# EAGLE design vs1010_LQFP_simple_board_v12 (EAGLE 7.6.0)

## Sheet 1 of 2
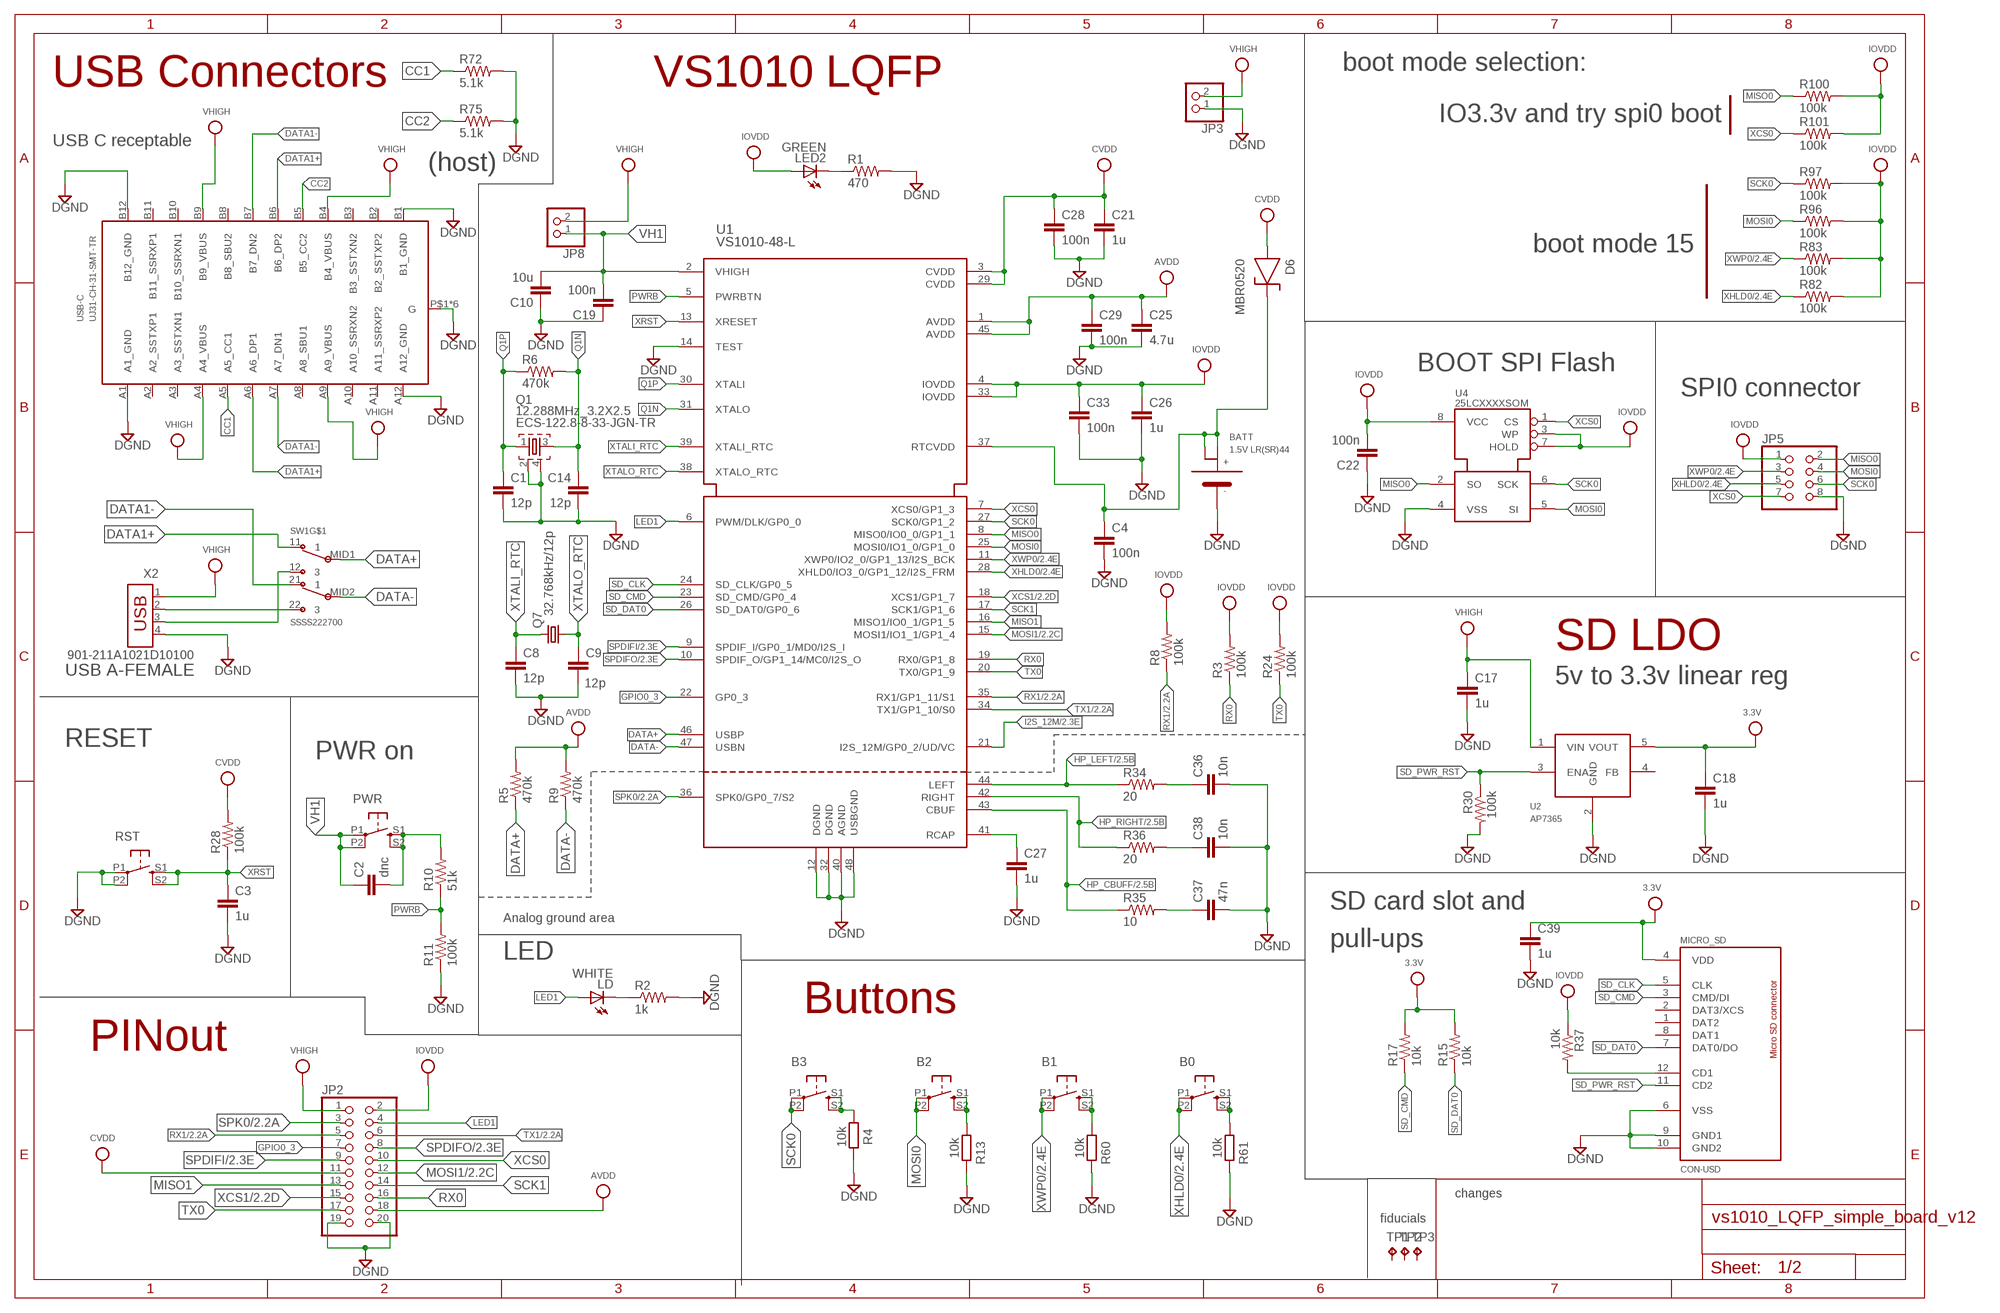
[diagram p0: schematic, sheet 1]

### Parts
B0  TS-1187A-C-E-B  SW_SMD-SW-4_5.1X5.1X2.5_TS-1187A-C-E-B_C318887  [SW_SMD-SW-4_5.1X5.1X2.5_TS-1187A-C-E-B_C318887]
B1  TS-1187A-C-E-B  SW_SMD-SW-4_5.1X5.1X2.5_TS-1187A-C-E-B_C318887  [SW_SMD-SW-4_5.1X5.1X2.5_TS-1187A-C-E-B_C318887]
B2  TS-1187A-C-E-B  SW_SMD-SW-4_5.1X5.1X2.5_TS-1187A-C-E-B_C318887  [SW_SMD-SW-4_5.1X5.1X2.5_TS-1187A-C-E-B_C318887]
B3  TS-1187A-C-E-B  SW_SMD-SW-4_5.1X5.1X2.5_TS-1187A-C-E-B_C318887  [SW_SMD-SW-4_5.1X5.1X2.5_TS-1187A-C-E-B_C318887]
BATT  1.5V LR(SR)44  BATT-LR44-TH  [KS2997]
C1  12p  C-EUC0603K  [C0603K]
C2  dnc  C-EUC0603K  [C0603K]
C3  1u  C-EUC0603K  [C0603K]
C4  100n  C-EUC0603K  [C0603K]
C8  12p  C-EUC0603K  [C0603K]
C9  12p  C-EUC0603K  [C0603K]
C10  10u  C-EUC0603K  [C0603K]
C14  12p  C-EUC0603K  [C0603K]
C17  1u  C-EUC0603K  [C0603K]
C18  1u  C-EUC0603K  [C0603K]
C19  100n  C-EUC0603K  [C0603K]
C21  1u  C-EUC0603K  [C0603K]
C22  100n  C-EUC0603K  [C0603K]
C25  4.7u  C-EUC0603K  [C0603K]
C26  1u  C-EUC0603K  [C0603K]
C27  1u  C-EUC0603K  [C0603K]
C28  100n  C-EUC0603K  [C0603K]
C29  100n  C-EUC0603K  [C0603K]
C33  100n  C-EUC0603K  [C0603K]
C36  10n  C-EUC0603K  [C0603K]
C37  47n  C-EUC0603K  [C0603K]
C38  10n  C-EUC0603K  [C0603K]
C39  1u  C-EUC0603K  [C0603K]
D6  MBR0520  [SOD-123]
JP2  PINHD-2X10  [2X10]
JP3  PINHD-1X2  [1X02]
JP5  PINHD-2X4  [2X04]
JP8  PINHD-1X2  [1X02]
LD  WHITE  LEDCHIP-LED0805  [CHIP-LED0805]
LED2  GREEN  LEDCHIP-LED0805  [CHIP-LED0805]
MICRO_SD  CON-USD  [MSSN09-A0-3000]
PWR  TS-1187A-C-E-B  SW_SMD-SW-4_5.1X5.1X2.5_TS-1187A-C-E-B_C318887  [SW_SMD-SW-4_5.1X5.1X2.5_TS-1187A-C-E-B_C318887]
Q1  12.288MHz_3.2X2.5  CRYSTAL_3.2X2.5  [3.2X2.5_CRYSTAL]
Q7  32.768kHz/12p  CRYSTAL3.2X1.5MM  [CRYSTAL_1206]
R1  470  R-US_R0603  [R0603]
R2  1k  R-US_R0603  [R0603]
R3  100k  R-US_R0603  [R0603]
R4  10k  R-EU_R0603  [R0603]
R5  470k  R-US_R0603  [R0603]
R6  470k  R-US_R0603  [R0603]
R8  100k  R-US_R0603  [R0603]
R9  470k  R-US_R0603  [R0603]
R10  51k  R-US_R0603  [R0603]
R11  100k  R-US_R0603  [R0603]
R13  10k  R-EU_R0603  [R0603]
R15  10k  R-US_R0603  [R0603]
R17  10k  R-US_R0603  [R0603]
R24  100k  R-US_R0603  [R0603]
R28  100k  R-US_R0603  [R0603]
R30  100k  R-US_R0603  [R0603]
R34  20  R-US_R0603  [R0603]
R35  10  R-US_R0603  [R0603]
R36  20  R-US_R0603  [R0603]
R37  10k  R-US_R0603  [R0603]
R60  10k  R-EU_R0603  [R0603]
R61  10k  R-EU_R0603  [R0603]
R72  5.1k  R-US_R0603  [R0603]
R75  5.1k  R-US_R0603  [R0603]
R82  100k  R-US_R0603  [R0603]
R83  100k  R-US_R0603  [R0603]
R96  100k  R-US_R0603  [R0603]
R97  100k  R-US_R0603  [R0603]
R100  100k  R-US_R0603  [R0603]
R101  100k  R-US_R0603  [R0603]
RST  TS-1187A-C-E-B  SW_SMD-SW-4_5.1X5.1X2.5_TS-1187A-C-E-B_C318887  [SW_SMD-SW-4_5.1X5.1X2.5_TS-1187A-C-E-B_C318887]
SW1  SSSS222700  SWITCH_ON-ON_DUAL_SSSS222700_C136144  [SWITCH_ON-ON_DUAL_SSSS222700_C136144]
TP1  TPTP10R  [TP10R]
TP2  TPTP10R  [TP10R]
TP3  TPTP10R  [TP10R]
U1  VS1010-48-L  [LQFP48]
U2  AP7365  [SOT23-5L]
U4  25LCXXXXSOM  [SO-8MN]
USB-C  UJ31-CH-31-SMT-TR  USB_C  [UJ31-CH-31-SMT-TR]
X2  901-211A1021D10100  USB-AH  [USB-S]

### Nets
3.3V: C18.1 C39.1 MICRO_SD.4(VDD) R15.2 R17.2 U2.5(VOUT)
AVDD: C25.1 C29.1 JP2.18 R5.2 R9.2 U1.1(AVDD) U1.45(AVDD) ; also sheet 2
CC1: R72.1 USB-C.A5(A5_CC1)
CC2: R75.1 USB-C.B5(B5_CC2)
CVDD: C21.1 C28.1 D6.ANODE JP2.11 R28.2 U1.3(CVDD) U1.29(CVDD)
DATA1+: SW1.11 USB-C.A6(A6_DP1) USB-C.B6(B6_DP2)
DATA1-: SW1.21 USB-C.A7(A7_DN1) USB-C.B7(B7_DN2)
DATA+: R5.1 SW1.MID1(MID) U1.46(USBP)
DATA-: R9.1 SW1.MID2(MID) U1.47(USBN)
DGND: BATT.NEG(-) C1.2 C3.2 C4.2 C8.2 C9.2 C10.1 C14.2 C17.2 C18.2 C19.1 C21.2 C22.1 C25.2 C26.2 C27.2 C28.2 C29.2 C33.2 C36.2 C37.2 C38.2 C39.2 JP2.19 JP2.20 JP3.1 JP5.8 MICRO_SD.6(VSS) MICRO_SD.9(GND1) MICRO_SD.10(GND2) Q1.2 Q1.4 R1.2 R2.2 R4.2 R11.1 R13.2 R30.2 R60.2 R61.2 R72.2 R75.2 RST.P1 RST.P2 U1.12(DGND) U1.14(TEST) U1.32(DGND) U1.40(AGND) U1.48(USBGND) U2.2(GND) U4.4(VSS) USB-C.A1(A1_GND) USB-C.A12(A12_GND) USB-C.B1(B1_GND) USB-C.B12(B12_GND) USB-C.P$1(G) USB-C.P$3(G) USB-C.P$4(G) USB-C.P$6(G) USB-C.P$7(G) USB-C.P$8(G) X2.4 ; also sheet 2
GPIO0_3: JP2.7 U1.22(GP0_3)
HP_CBUFF: R35.1 U1.43(CBUF) ; also sheet 2
HP_LEFT: R34.1 U1.44(LEFT) ; also sheet 2
HP_RIGHT: R36.1 U1.42(RIGHT) ; also sheet 2
I2S_12M: U1.21(I2S_12M/GP0_2/UD/VC) ; also sheet 2
IOVDD: C22.2 C26.1 C33.1 JP2.2 JP5.1 LED2.A R3.2 R8.2 R24.2 R37.1 R82.2 R83.2 R96.2 R97.2 R100.2 R101.2 U1.4(IOVDD) U1.33(IOVDD) U4.3(WP) U4.7(HOLD) U4.8(VCC) ; also sheet 2
LED1: JP2.4 LD.A U1.6(PWM/DLK/GP0_0)
MISO0: JP5.2 R100.1 U1.8(MISO0/IO0_0/GP1_1) U4.2(SO)
MISO1: JP2.13 U1.16(MISO1/IO0_1/GP1_5)
MOSI0: B2.P1 B2.P2 JP5.4 R96.1 U1.25(MOSI0/IO1_0/GP1_0) U4.5(SI)
MOSI1: JP2.12 U1.15(MOSI1/IO1_1/GP1_4) ; also sheet 2
N$2: LD.C R2.1
N$3: LED2.C R1.1
N$6: B1.S1 B1.S2 R60.1
N$9: C2.2 PWR.S1 PWR.S2 R10.2
N$10: C27.1 U1.41(RCAP)
N$17: C36.1 R34.2
N$19: C38.1 R36.2
N$20: C37.1 R35.2
N$21: MICRO_SD.12(CD1) R37.2
N$41: B0.S1 B0.S2 R61.1
N$89: B2.S1 B2.S2 R13.1
N$100: B3.S1 B3.S2 R4.1
PWRB: R10.1 R11.2 U1.5(PWRBTN)
Q1N: C14.1 Q1.3 R6.2 U1.31(XTALO)
Q1P: C1.1 Q1.1 R6.1 U1.30(XTALI)
RTCVDD: BATT.P1(+) BATT.P2(+1) C4.1 D6.CATHODE U1.37(RTCVDD)
RX0: JP2.16 R3.1 U1.19(RX0/GP1_8)
RX1: JP2.5 R8.1 U1.35(RX1/GP1_11/S1) ; also sheet 2
SCK0: B3.P1 B3.P2 JP5.6 R97.1 U1.27(SCK0/GP1_2) U4.6(SCK)
SCK1: JP2.14 U1.17(SCK1/GP1_6)
SD_CLK: MICRO_SD.5(CLK) U1.24(SD_CLK/GP0_5)
SD_CMD: MICRO_SD.3(CMD/DI) R17.1 U1.23(SD_CMD/GP0_4)
SD_DAT0: MICRO_SD.7(DAT0/DO) R15.1 U1.26(SD_DAT0/GP0_6)
SD_PWR_RST: MICRO_SD.11(CD2) R30.1 U2.3(ENA)
SPDIFI: JP2.9 U1.9(SPDIF_I/GP0_1/MD0/I2S_I) ; also sheet 2
SPDIFO: JP2.8 U1.10(SPDIF_O/GP1_14/MC0/I2S_O) ; also sheet 2
SPK0: JP2.3 U1.36(SPK0/GP0_7/S2) ; also sheet 2
TX0: JP2.17 R24.1 U1.20(TX0/GP1_9)
TX1: JP2.6 U1.34(TX1/GP1_10/S0) ; also sheet 2
USB2+: SW1.12 X2.3
USB2-: SW1.22 X2.2
VH1: C2.1 C10.2 C19.2 JP8.1 PWR.P1 PWR.P2 U1.2(VHIGH)
VHIGH: C17.1 JP2.1 JP3.2 JP8.2 U2.1(VIN) USB-C.A4(A4_VBUS) USB-C.A9(A9_VBUS) USB-C.B4(B4_VBUS) USB-C.B9(B9_VBUS) X2.1
XCS0: JP2.10 JP5.7 R101.1 U1.7(XCS0/GP1_3) U4.1(CS)
XCS1: JP2.15 U1.18(XCS1/GP1_7) ; also sheet 2
XHLD0: B0.P1 B0.P2 JP5.5 R82.1 U1.28(XHLD0/IO3_0/GP1_12/I2S_FRM) ; also sheet 2
XRST: C3.1 R28.1 RST.S1 RST.S2 U1.13(XRESET)
XTALI_RTC: C8.1 Q7.2 U1.39(XTALI_RTC)
XTALO_RTC: C9.1 Q7.1 U1.38(XTALO_RTC)
XWP0: B1.P1 B1.P2 JP5.3 R83.1 U1.11(XWP0/IO2_0/GP1_13/I2S_BCK) ; also sheet 2
Unconnected: MICRO_SD.1(DAT2) MICRO_SD.2(DAT3/XCS) MICRO_SD.8(DAT1) TP1.TP TP2.TP TP3.TP U2.4(FB) USB-C.A2(A2_SSTXP1) USB-C.A3(A3_SSTXN1) USB-C.A8(A8_SBU1) USB-C.A10(A10_SSRXN2) USB-C.A11(A11_SSRXP2) USB-C.B2(B2_SSTXP2) USB-C.B3(B3_SSTXN2) USB-C.B8(B8_SBU2) USB-C.B10(B10_SSRXN1) USB-C.B11(B11_SSRXP1)

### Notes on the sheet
- USB Connectors | VS1010 LQFP | boot mode selection:
- IO3.3v and try spi0 boot
- USB C receptable
- (host)
- boot mode 15
- BOOT SPI Flash
- SPI0 connector
- SD LDO
- USB A-FEMALE
- 5v to 3.3v linear reg
- RESET
- PWR on
- SD card slot and
- Analog ground area
- pull-ups
- LED
- Buttons
- PINout
- changes
- fiducials

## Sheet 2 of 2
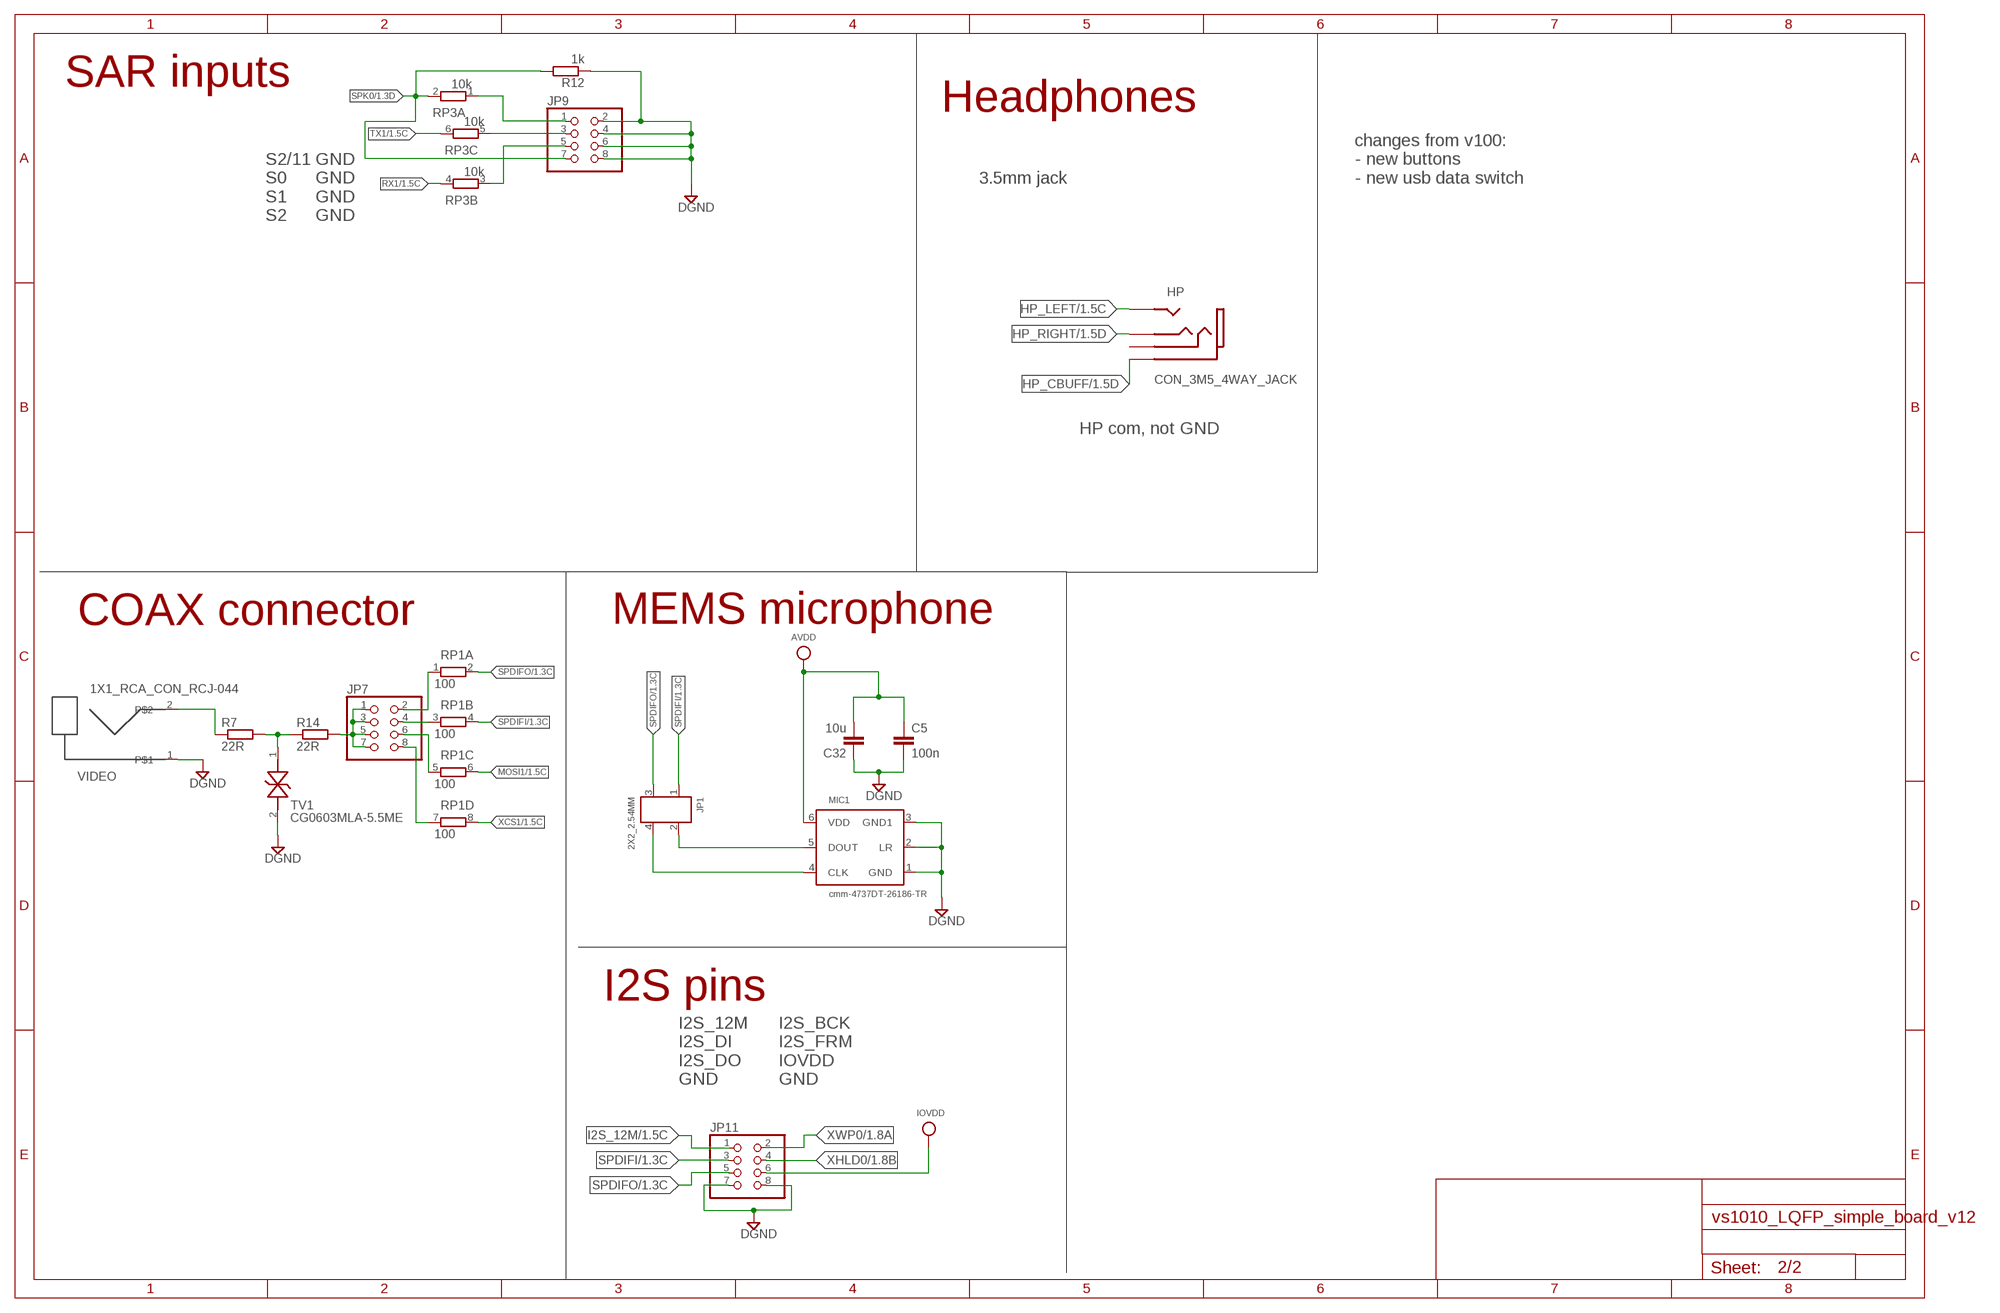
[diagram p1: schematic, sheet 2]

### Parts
C5  100n  C-EUC0603K  [C0603K]
C32  10u  C-EUC0805  [C0805]
HP  CON_3M5_4WAY_JACK  CON_3M5_4WAY_JACK-TH  [SJ-43514]
JP1  2X2_2.54MM  2X2_2.54MM_CON_THRU  [2X2_2.54MM_CON_THRU]
JP7  PINHD-2X4  [2X04]
JP9  PINHD-2X4  [2X04]
JP11  PINHD-2X4  [2X04]
MIC1  cmm-4737DT-26186-TR  MEMS_MIC_CMM-4737DT-26186-TR  [MIC_MEMS_CMM-4737DT]
R7  22R  R-EU_R0603  [R0603]
R12  1k  R-EU_R0603  [R0603]
R14  22R  R-EU_R0603  [R0603]
RP1  100  RESPAK-4X1206  [RAS_ARR_1206]
RP3  10k  RESPAK-4X1206  [RAS_ARR_1206]
TV1  CG0603MLA-5.5ME  [0603]
VIDEO  1X1_RCA_CON_RCJ-044  [1X1_RCA_CON_RCJ-044]

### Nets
AVDD: C5.1 C32.2 MIC1.6(VDD) ; also sheet 1
DGND: C5.2 C32.1 JP9.2 JP9.4 JP9.6 JP9.8 JP11.7 JP11.8 MIC1.1(GND) MIC1.2(LR) MIC1.3(GND1) R12.1 TV1.2(A2) VIDEO.1 ; also sheet 1
HP_CBUFF: HP.5(GND) ; also sheet 1
HP_LEFT: HP.4(LEFT) ; also sheet 1
HP_RIGHT: HP.1(RIGHT) ; also sheet 1
I2S_12M: JP11.1 ; also sheet 1
IOVDD: JP11.6 ; also sheet 1
MOSI1: RP1.6 ; also sheet 1
N$5: JP9.3 RP3.5
N$7: JP9.5 RP3.3
N$8: JP1.2 MIC1.5(DOUT)
N$11: JP1.4 MIC1.4(CLK)
N$12: JP7.2 RP1.1
N$13: JP7.6 RP1.5
N$14: JP7.1 JP7.3 JP7.5 JP7.7 R14.2
N$15: JP7.4 RP1.3
N$16: JP7.8 RP1.7
N$18: R7.1 VIDEO.2
N$25: JP9.1 RP3.1
N$52: R7.2 R14.1 TV1.1(A1)
RX1: RP3.4 ; also sheet 1
SPDIFI: JP1.1 JP11.3 RP1.4 ; also sheet 1
SPDIFO: JP1.3 JP11.5 RP1.2 ; also sheet 1
SPK0: JP9.7 R12.2 RP3.2 ; also sheet 1
TX1: RP3.6 ; also sheet 1
XCS1: RP1.8 ; also sheet 1
XHLD0: JP11.4 ; also sheet 1
XWP0: JP11.2 ; also sheet 1
Unconnected: HP.6(POLE4) RP3.7 RP3.8

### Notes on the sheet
- SAR inputs
- Headphones
- 3.5mm jack
- changes from v100:
  - new buttons
  - new usb data switch
- S2/11
  S0   
  S1
  S2
- GND
  GND
  GND
  GND
- HP com, not GND
- COAX connector | MEMS microphone
- I2S pins
- I2S_12M 
  I2S_DI    
  I2S_DO 
  GND
- I2S_BCK
  I2S_FRM
  IOVDD
  GND

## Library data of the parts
B0 B1-B3 PWR RST = 121_PanunKomponentit:SW_SMD-SW-4_5.1X5.1X2.5_TS-1187A-C-E-B_C318887
BATT = Omat:BATT-LR44
C1-C5 C8-C10 C14 C17-C19 C21 C22 C25-C29 C33 C36-C39 = resistor:C-EU: CAPACITOR, European symbol
C32 = rcl:C-EU: CAPACITOR, European symbol
D6 = 121_PanunKomponentit:MBR0520
HP = Samin_e7:CON_3M5_4WAY_JACK
JP1 = 121_PanunKomponentit:2X2_2.54MM_CON_THRU
JP2 = pinhead:PINHD-2X10: PIN HEADER
JP3 JP8 = pinhead:PINHD-1X2: PIN HEADER
JP5 JP7 JP9 JP11 = pinhead:PINHD-2X4: PIN HEADER
LD LED2 = led:LED: LED
MIC1 = 121_PanunKomponentit:MEMS_MIC_CMM-4737DT-26186-TR
MICRO_SD = 114SaminOmat:CON-USD: Micro SD connector
Q1 = 121_PanunKomponentit:CRYSTAL_3.2X2.5
Q7 = antimode_x4:CRYSTAL: CRYSTAL
R1-R3 R5 R6 R8-R11 R15 R17 R24 R28 R30 R34-R37 R72 R75 R82 R83 R96 R97 R100 R101 = resistor:R-US_: RESISTOR, American symbol
R4 R7 R12-R14 R60 R61 = rcl:R-EU_: RESISTOR, European symbol
RP1 RP3 = Samin_e7:RESPAK-4X1206
SW1 = 121_PanunKomponentit:SWITCH_ON-ON_DUAL_SSSS222700_C136144
TP1-TP3 = testpad:TP: Test pad
TV1 = SaminOmat:CG0603MLA-5.5ME: Transient voltage suppressor
U1 = 121_PanunKomponentit:VS1010-48
U2 = HannunOmat:AP7365
U4 = 121_PanunKomponentit:25LCXXXX
USB-C = 121_PanunKomponentit:USB_C
VIDEO = 121_PanunKomponentit:1X1_RCA_CON_RCJ-044
X2 = SaminOmat:USB-A: AMP connector

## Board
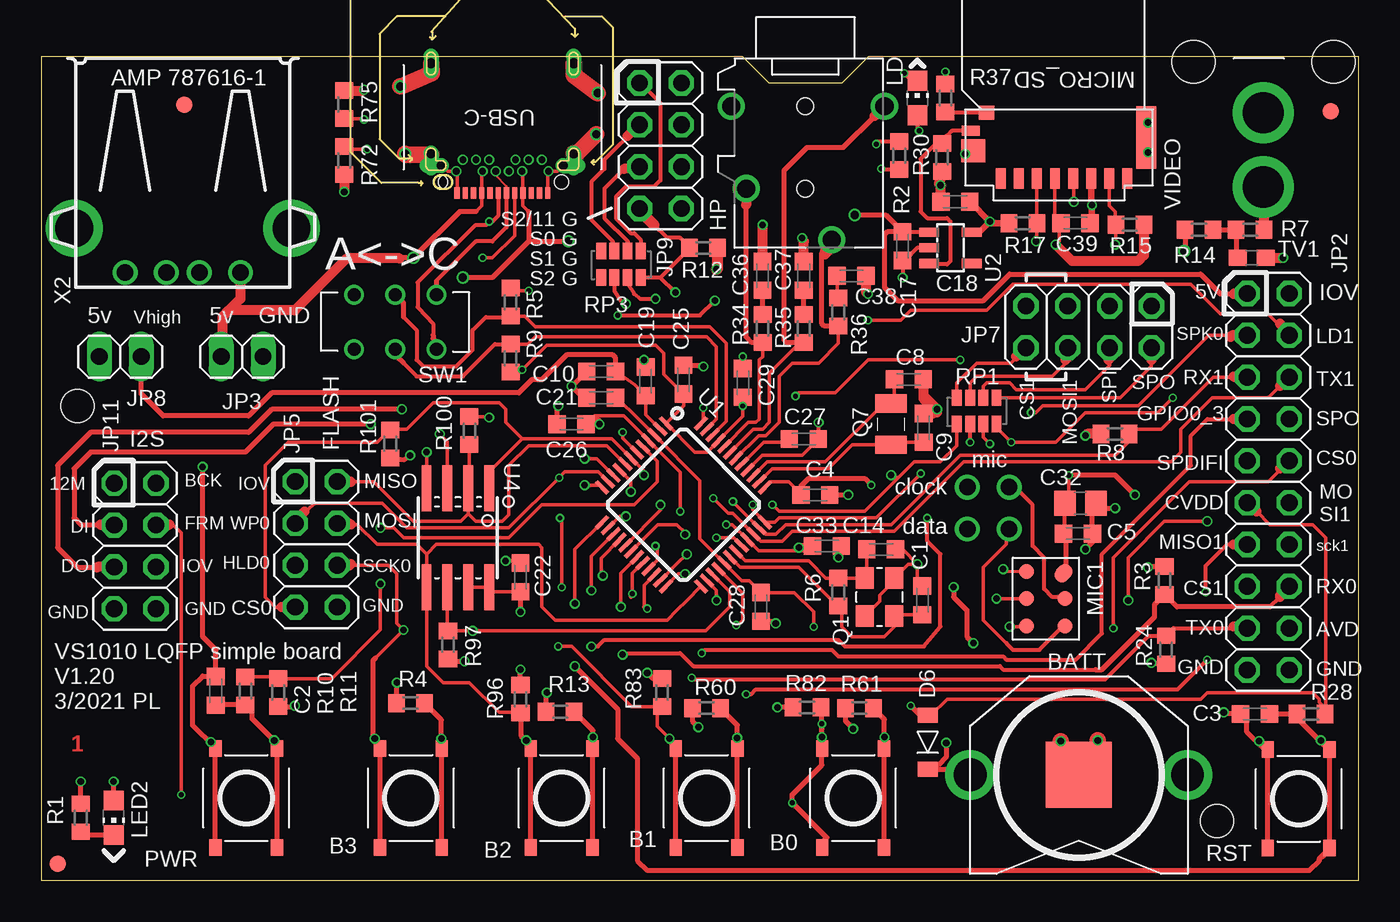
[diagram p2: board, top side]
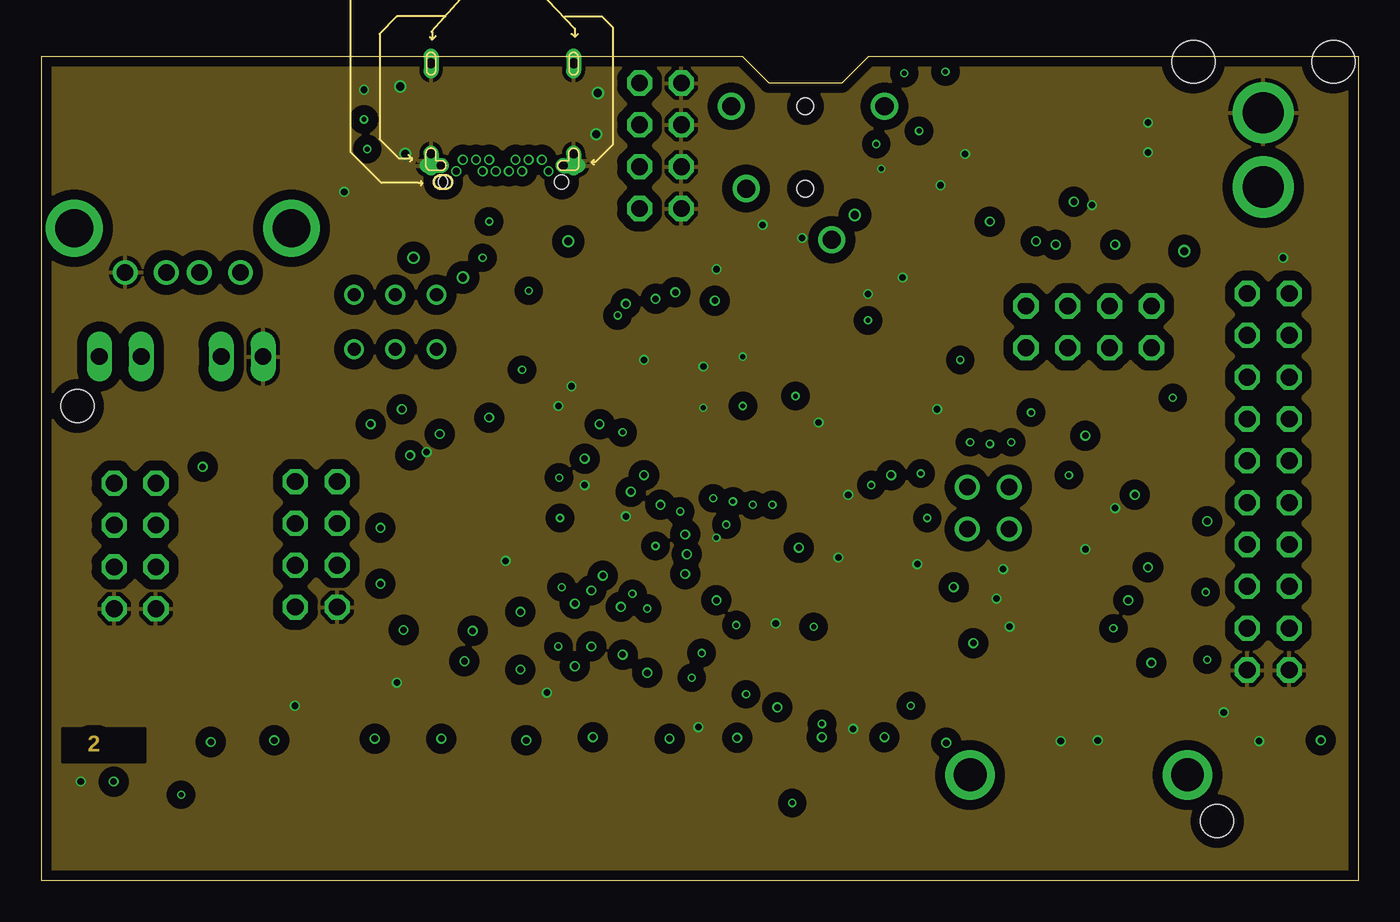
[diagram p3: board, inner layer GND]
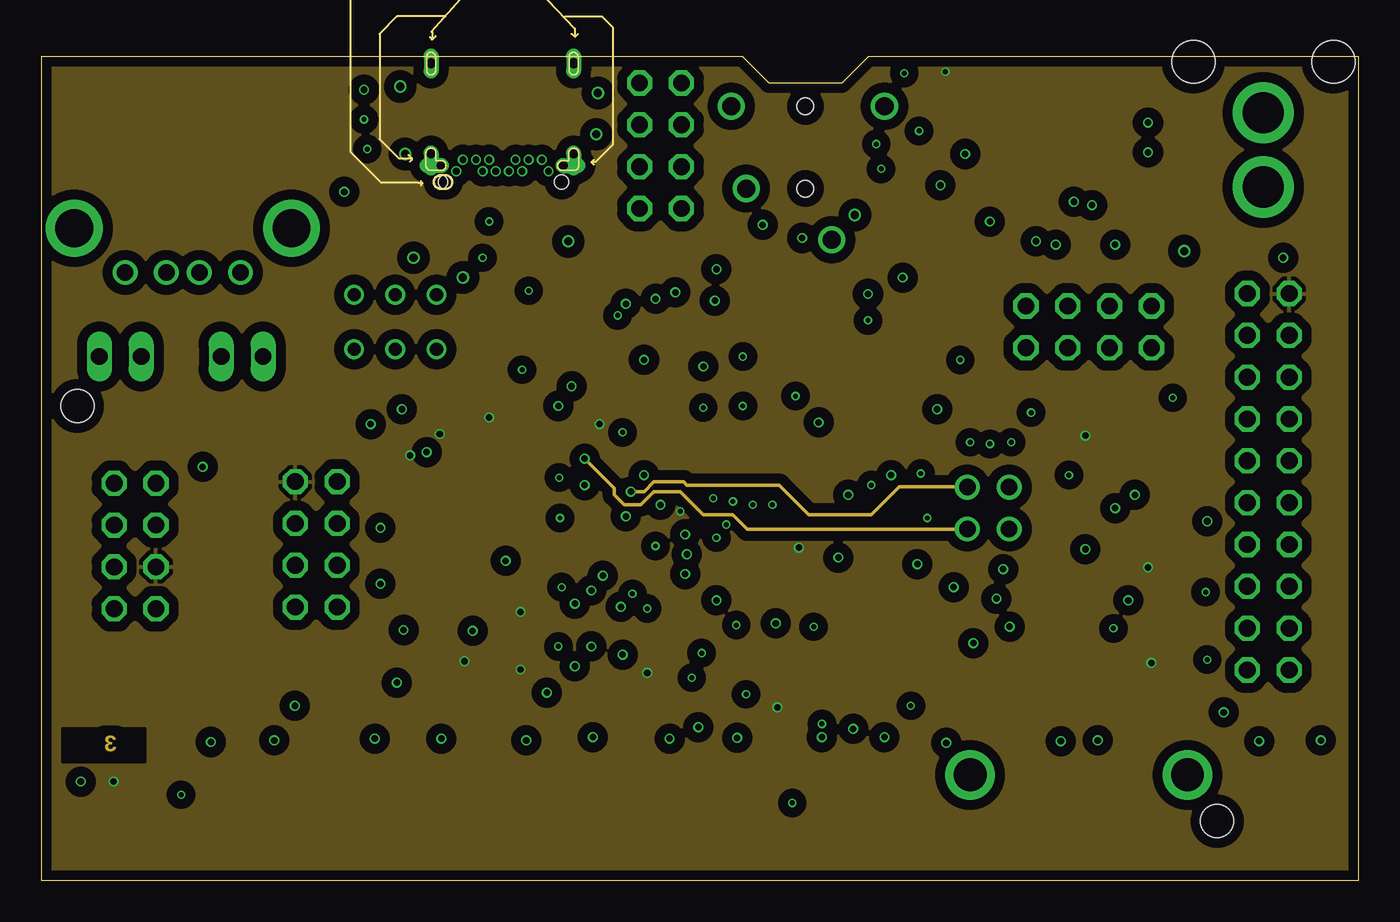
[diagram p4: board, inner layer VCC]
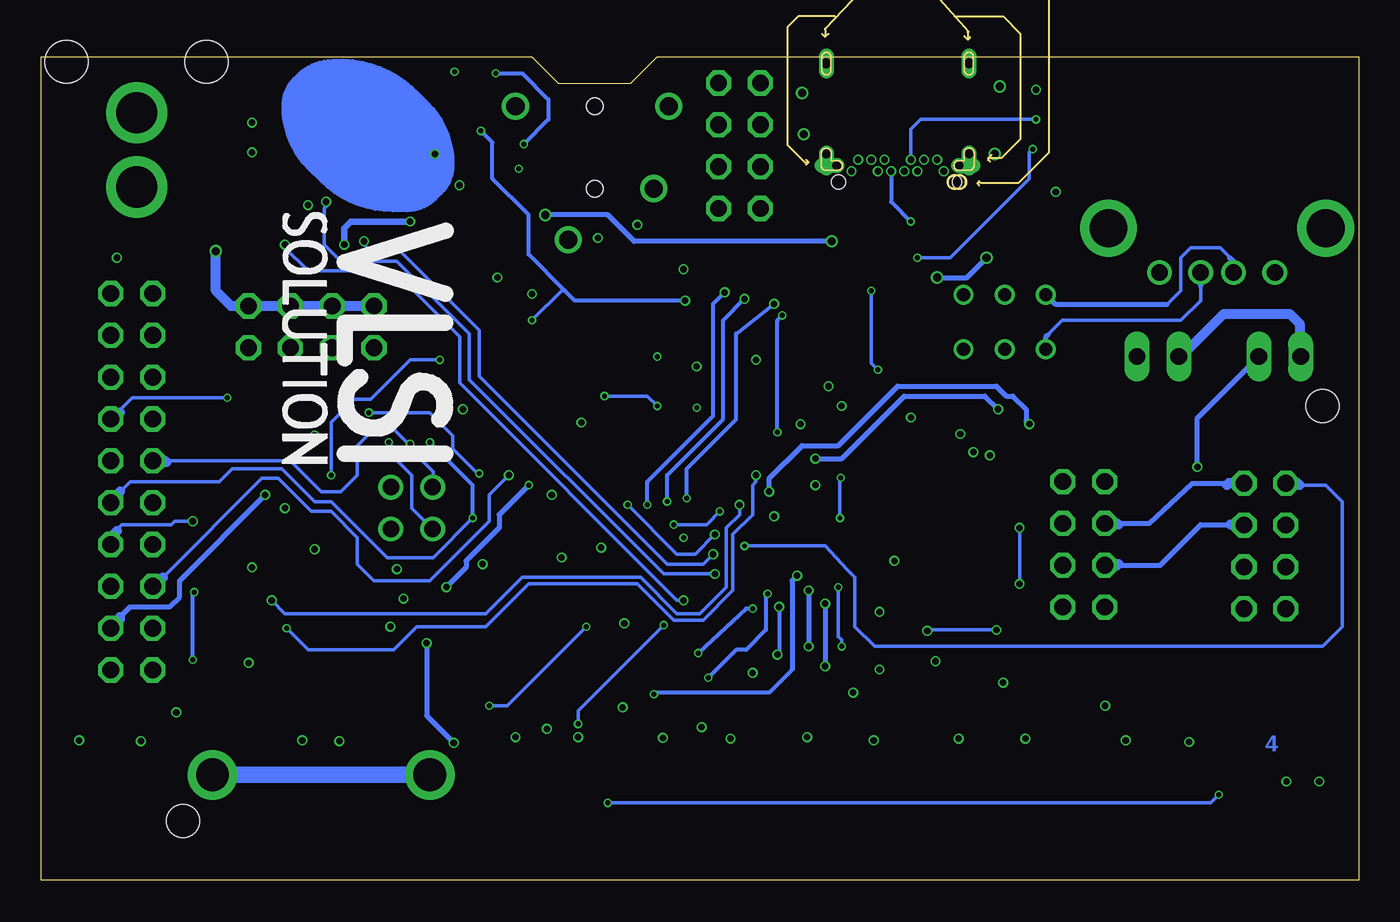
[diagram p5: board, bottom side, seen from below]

Size 80 x 50 mm. Coordinates in mm from the lower left corner, seen from the top.
Outline: 0,0 80,0 80,50 50.2,50 48.6,48.4 44.2,48.4 42.6,50 0,50 0,0
Copper layers (1*2+15*16): Top 0.035mm / dielectric 0.12mm / GND 0.0175mm / dielectric 1.2mm / VCC 0.0175mm / dielectric 0.12mm / Bottom 0.035mm
Design rules "4L_Smart_prototyping_usb-c_Eagle Rule": minimum track width 6mil, minimum drill 0.3mm, track to track 6mil, track to pad 6mil, pad to pad 6mil, via to via 6mil, smd to smd 0mil, copper to edge 6mil, drill to drill 12mil, minimum pad ring 0.1mm, minimum via ring 4mil, stop-mask expansion 2mil, vias tented up to drill 25mil, thermal gap 10mil
Holes 2 mm at 2.2,28.8 71.4,3.6

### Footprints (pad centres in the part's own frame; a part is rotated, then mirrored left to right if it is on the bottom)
SW_SMD-SW-4_5.1X5.1X2.5_TS-1187A-C-E-B_C318887 = smd 1 x 0.75: P1 -3,1.875; P2 3,1.875; S1 -3,-1.875; S2 3,-1.875
KS2997 = smd 4 x 4: NEG 0,0 | drill 2: P1 -6.6,0; P2 6.6,0
C0603K = smd 1.05 x 1.08: 1 -0.875,0; 2 0.875,0
C0805 = smd 1.3 x 1.5: 1 -0.95,0; 2 0.95,0
SOD-123 = smd 0.914 x 1.219: ANODE -1.638,0; CATHODE 1.638,0
SJ-43514 = drill 1.1: 1 8.1,1.6; 4 5,-3.6; 5 0,4.8; 6 0,-4.5 | hole 1: 0,0; 5,0
2X2_2.54MM_CON_THRU = drill 1: 1 -1.27,1.27; 2 1.27,1.27; 3 -1.27,-1.27; 4 1.27,-1.27
2X10 = drill 1.016 octagon: 1 -11.43,-1.27; 2 -11.43,1.27; 3 -8.89,-1.27; 4 -8.89,1.27; 5 -6.35,-1.27; 6 -6.35,1.27; 7 -3.81,-1.27; 8 -3.81,1.27; 9 -1.27,-1.27; 10 -1.27,1.27; 11 1.27,-1.27; 12 1.27,1.27; 13 3.81,-1.27; 14 3.81,1.27; 15 6.35,-1.27; 16 6.35,1.27; 17 8.89,-1.27; 18 8.89,1.27; 19 11.43,-1.27; 20 11.43,1.27
1X02 = drill 1.016 long: 1 -1.27,0; 2 1.27,0
2X04 = drill 1.016 octagon: 1 -3.81,-1.27; 2 -3.81,1.27; 3 -1.27,-1.27; 4 -1.27,1.27; 5 1.27,-1.27; 6 1.27,1.27; 7 3.81,-1.27; 8 3.81,1.27
CHIP-LED0805 = smd 1.2 x 1.2: A 0,-1.05; C 0,1.05
MIC_MEMS_CMM-4737DT = smd 0.91 x 0.91: 1 -1.17,1.65; 2 -1.17,0; 3 -1.17,-1.65; 4 1.17,-1.65; 5 1.17,0 | smd 1.2 x 0.91 rotated 45: 6 1.07,1.55
MSSN09-A0-3000 = smd 0.6 x 1.25: 1 3.85,0; 2 2.75,0; 3 1.65,0; 4 0.55,0; 5 -0.55,0; 6 -1.65,0; 7 -2.75,0; 8 -3.85,0 | smd 1.2 x 3.79: 9 -5,-2.5 | smd 1.45 x 1.4: 10 5.5,-1.7 | smd 1.1 x 0.6: 11 5.65,-2.9 | smd 0.95 x 0.85: 12 4.7,-4
3.2X2.5_CRYSTAL = smd 1.3 x 1.1: 1 -1.15,-0.9; 2 1.15,-0.9; 3 1.15,0.9; 4 -1.15,0.9
CRYSTAL_1206 = smd 1.1 x 1.9: 1 -1.25,0; 2 1.25,0
R0603 = smd 1 x 1.1: 1 -0.85,0; 2 0.85,0
RAS_ARR_1206 = smd 1 x 0.6: 1 -0.8,1.2; 2 0.8,1.2; 3 -0.8,0.4; 4 0.8,0.4; 5 -0.8,-0.4; 6 0.8,-0.4; 7 -0.8,-1.2; 8 0.8,-1.2
SWITCH_ON-ON_DUAL_SSSS222700_C136144 = drill 0.8: 11 -2.5,-1.65; 12 2.5,-1.65; 21 -2.5,1.65; 22 2.5,1.65; MID1 0,-1.65; MID2 0,1.65
TP10R = smd 1 x 1: TP 0,0
0603 = smd 1.1 x 1: 1 -0.85,0; 2 0.85,0
LQFP48 = smd 0.25 x 1: 1 -2.75,-4.25; 2 -2.25,-4.25; 3 -1.75,-4.25; 4 -1.25,-4.25; 5 -0.75,-4.25; 6 -0.25,-4.25; 7 0.25,-4.25; 8 0.75,-4.25; 9 1.25,-4.25; 10 1.75,-4.25; 11 2.25,-4.25; 12 2.75,-4.25; 25 2.75,4.25; 26 2.25,4.25; 27 1.75,4.25; 28 1.25,4.25; 29 0.75,4.25; 30 0.25,4.25; 31 -0.25,4.25; 32 -0.75,4.25; 33 -1.25,4.25; 34 -1.75,4.25; 35 -2.25,4.25; 36 -2.75,4.25 | smd 1 x 0.25: 13 4.25,-2.75; 14 4.25,-2.25; 15 4.25,-1.75; 16 4.25,-1.25; 17 4.25,-0.75; 18 4.25,-0.25; 19 4.25,0.25; 20 4.25,0.75; 21 4.25,1.25; 22 4.25,1.75; 23 4.25,2.25; 24 4.25,2.75; 37 -4.25,2.75; 38 -4.25,2.25; 39 -4.25,1.75; 40 -4.25,1.25; 41 -4.25,0.75; 42 -4.25,0.25; 43 -4.25,-0.25; 44 -4.25,-0.75; 45 -4.25,-1.25; 46 -4.25,-1.75; 47 -4.25,-2.25; 48 -4.25,-2.75
SOT23-5L = smd 0.55 x 1.2: 1 -0.95,-1.3; 2 0,-1.3; 3 0.95,-1.3; 4 0.95,1.3; 5 -0.95,1.3
SO-8MN = smd 0.6 x 2.8: 1 -1.905,-3.013; 2 -0.635,-3.013; 3 0.635,-3.013; 4 1.905,-3.013; 5 1.905,3.013; 6 0.635,3.013; 7 -0.635,3.013; 8 -1.905,3.013
UJ31-CH-31-SMT-TR = smd 0.32 x 0.7: A1 -2.75,0.66; A2 -2.25,0.66; A3 -1.75,0.66; A4 -1.25,0.66; A5 -0.75,0.66; A6 -0.25,0.66; A7 0.25,0.66; A8 0.75,0.66; A9 1.25,0.66; A10 1.75,0.66; A11 2.25,0.66; A12 2.75,0.66 | drill 0.4 pad 0.6: B1 2.8,-0.65; B2 2.4,-1.35; B3 1.6,-1.35; B4 1.2,-0.65; B5 0.8,-1.35; B6 0.4,-0.65; B7 -0.4,-0.65; B8 -0.8,-1.35; B9 -1.2,-0.65; B10 -1.6,-1.35; B11 -2.4,-1.35; B12 -2.8,-0.65 | drill 0.6 pad 0.8 offset: P$1 -3.68,-1; P$3 -4.33,-1.75; P$4 3.68,-1; P$6 4.33,-1.75 | drill 0.6 pad 0.9 long: P$7 -4.33,-7.2; P$8 4.33,-7.2 | hole 0.85: 3.45,0; -3.6,0; 3.75,0
1X1_RCA_CON_RCJ-044 = drill 2.5: 1 -4,0; 2 -8.5,0 | hole 2.6: -0.9,4.25; -0.9,-4.25
USB-S = drill 1: 1 -3.5,12.99; 2 -1,12.99; 3 1,12.99; 4 3.5,12.99 | drill 2.3: P$1 -6.6,10.3; P$2 6.6,10.3

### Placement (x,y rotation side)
B0  49.3,5 90 top
B1  40.4,5 90 top
B2  31.6,5 90 top
B3  22.45,5 90 top
BATT  63,6.4 180 top
C1  53.5,17 90 top
C2  10.6,11.5 270 top
C3  73.7,10.1 180 top
C4  47,23.4 0 top
C5  62.95,21.05 0 top
C8  52.68,30.42 0 top
C9  53.58,27.47 90 top
C10  34,30.9 0 top
C14  51,20.1 0 top
C17  52.3,38.5 270 top
C18  55.5,41.2 180 top
C19  36.7,30.3 270 top
C21  34,29.3 180 top
C22  29.1,18.4 270 top
C25  39,30.4 90 top
C26  32.2,27.7 180 top
C27  46.3,26.8 0 top
C28  43.7,16.6 270 top
C29  42.6,30.2 90 top
C32  63.1,22.9 180 top
C33  47.7,20.3 0 top
C36  43.8,36.7 90 top
C37  46.3,36.7 90 top
C38  49.2,36.7 0 top
C39  62.8,39.9 0 top
D6  53.83,8.38 270 top
HP  46.4,47 270 top
JP1  57.5,22.6 0 top
JP2  74.5,24.2 270 top
JP3  12.2,31.8 180 top
JP5  16.7,20.4 270 top
JP7  63.6,33.6 180 top
JP8  4.8,31.8 180 top
JP9  37.6,44.6 270 top
JP11  5.7,20.3 270 top
LD  53.2,47.5 0 top
LED2  4.4,3.8 180 top
MIC1  61,17.1 0 top
MICRO_SD  62.1,42.6 180 top
PWR  12.45,5 90 top
Q1  50.9,17.2 90 top
Q7  51.59,27.7 90 top
R1  2.4,3.8 90 top
R2  52.1,44 270 top
R3  68.2,18.2 90 top
R4  22.43,10.76 180 top
R5  28.5,35.1 90 top
R6  48.4,17.5 90 top
R7  73.4,39.5 180 top
R8  65.2,27.1 180 top
R9  28.5,31.7 270 top
R10  12.4,11.5 270 top
R11  14.4,11.4 90 top
R12  40.2,38.4 180 top
R13  31.51,10.24 180 top
R14  70.3,39.5 180 top
R15  66.1,39.8 0 top
R17  59.6,39.9 180 top
R24  68.3,14 270 top
R28  77.1,10.1 0 top
R30  54.7,43.9 270 top
R34  43.8,33.5 90 top
R35  46.3,33.5 90 top
R36  48.4,34.5 90 top
R37  54.9,47.5 270 top
R60  40.39,10.46 180 top
R61  49.67,10.46 180 top
R72  18.4,43.7 270 top
R75  18.4,47.1 90 top
R82  46.5,10.5 180 top
R83  37.7,11.4 90 top
R96  29.1,11 90 top
R97  24.7,14.3 270 top
R100  26,27.3 90 top
R101  21.2,26.5 270 top
RP1  56.8,28.5 270 top
RP3  35.2,37.4 270 top
RST  76.35,4.95 90 top
SW1  21.5,33.9 180 top
TP1  1,1 0 top
TP2  78.3,46.7 0 top
TP3  8.7,47.1 0 top
TV1  73.5,37.8 0 top
U1  39,22.8 225 top
U2  55.2,38.4 270 top
U4  25.3,20.8 180 top
U$2  [LOGO]  65.7,50.1 270 bottom
USB-C  28,42.4 180 top
VIDEO  74.2,50.6 90 top
X2  8.6,49.9 180 top

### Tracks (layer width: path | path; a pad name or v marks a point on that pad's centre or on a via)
3.3V  (via drill 0.4)
  Top 0.2: MICRO_SD.4 61.55,40.27 C39.1 61.8,39.77 61.8,38.8 v61.6,38.6 | U2.5 56.95,39.35
  Top 0.4: 56.95,39.35 v57.6,40 | R17.2 57.7,39.9 v57.6,40 | C18.1 56.4,41.2 v57.6,40
  Top 0.6: R15.2 66.95,37.95 66.6,37.6 62.6,37.6 v61.6,38.6
  Bottom 0.4: v61.6,38.6 61.6,39.6 61.2,40 v57.6,40
AVDD  (via drill 0.3, 0.4)
  Top 0.2: C29.1 v42.6,28.8 42.6,28.17 U1.45 40.43,26 39.69,26 U1.1 38.79,28.6 39,28.8 C25.1 37.8,30.73 37.8,32 37.3,32.5 30.7,32.5 v29.2,31 | v29.2,31 29.05,30.85 28.73,30.85 | 28.73,30.85 R9.2 | 28.73,30.85 28.88,31 v29.2,31 | R5.2 28.65,35.8 v29.6,35.8 | v45.8,29.4 46,29.6 48.2,29.6 50.2,31.6 v55.8,31.6 | v62.4,24.6 62.4,23.15 C32.2
  Top 0.25: MIC1.6 62.25,18.83 | 62.15,21.2 C32.2
  Top 0.3: v66.4,23.4 65.2,24.6 v62.4,24.6 | 62.25,18.83 62.25,20.88 C5.1 62.08,21.12 62.15,21.2
  Bottom 0.2: v29.2,31 29.6,31.4 v29.6,35.8 | v42.6,28.8 43.2,29.4 v45.8,29.4 | v55.8,31.6 57.6,31.6 60,29.2 61,29.2 62.4,27.8 v62.4,24.6
  Bottom 0.3: JP2.18 75.77,15.43 75.2,16 74.6,16.6 72.2,16.6 71.6,17.2 71.6,18.2 v66.4,23.4
  Bottom 0.6: JP2.18 75.2,15.88 75.2,16
CC1  (via drill 0.3)
  Top 0.2: USB-C.A5 28.75,39.15 27.4,37.8 v26.8,37.8 | v19.8,44.4 18.55,44.4 R72.1
  Bottom 0.2: v26.8,37.8 24.8,37.8 20,42.6 20,44.2 v19.8,44.4
CC2  (via drill 0.3)
  Top 0.2: R75.1 19.55,46.25 v19.6,46.2
  Bottom 0.2: USB-C.B5 27.2,45.6 26.6,46.2 v19.6,46.2
CVDD  (via drill 0.3)
  Top 0.2: C21.1 35.77,28.5 U1.3 40,24.27 40,20.74 U1.29 42.54,18.2 43,18.2 43.7,17.5 C28.1 45.73,17.48 46.9,16.3 v46.9,15.4 | R28.2 78,10.15 78,10.4 | 78,10.4 78,20.8 77.2,21.6 74.6,21.6 73.8,22.4 | 73.4,22.8 73.27,22.93 JP2.11 | D6.ANODE 54.02,10.02 55,11 70.4,11 70.8,11.4 77.2,11.4 77.6,11 77.6,10.8 78,10.4
  Top 0.3: D6.ANODE 53.38,10.02 v52.8,10.6
  Top 0.6: 73.4,22.8 73.8,22.4
  Bottom 0.2: v46.9,15.4 51.7,10.6 v52.8,10.6
DATA1+
  Top 0.152: USB-C.B6 27.6,42.8 28.25,42.15 USB-C.A6
  Top 0.25: USB-C.A6 28.25,39.65 27.4,38.8 26.4,38.8 24,36.4
  Top 0.3: 24,36.4 SW1.11
DATA1-  (via drill 0.3)
  Top 0.25: USB-C.A7 27.75,40.35 27.4,40 v27.2,40 27,39.8 26.4,39.8 22.85,36.3 22.85,34.8 23.8,33.8 23.8,33.1
  Top 0.3: 23.8,33.1 23.8,32.9 SW1.21
  Bottom 0.25: USB-C.B7 28.4,41.2 v27.2,40
DATA+
  Top 0.2: U1.46 41.6,27.88 41.6,32.6 40.6,33.6 30,33.6 29.35,34.25 R5.1
  Top 0.25: 22,34.2 22.8,33.4 22.8,31.6 23.2,31.2 25.2,31.2 26.2,32.2 26.2,33.4 27,34.2 28.45,34.2 R5.1
  Top 0.3: 22,34.2 22,35.05 SW1.MID1
DATA-
  Top 0.2: U1.47 41,27.98 41,32.4 40.4,33 30,33 29.55,32.55 R9.1
  Top 0.25: 22,31.4 22.8,30.6 25.6,30.6 27.55,32.55 R9.1
  Top 0.3: 22,31.4 21.6,31.8 21.6,32.15 SW1.MID2
DGND  (via drill 0.3, 0.4, 0.5)
  Top 0.2: U1.48 40.2,27.89 v40.2,28.7 | C29.2 v42.6,31.8 | U1.40 43.77,25.8 46.2,25.8 47,26.6 47.17,26.77 C27.2 | U1.32 42.06,20.8 v41,20.8 | Q1.4 50.9,16.95 50.9,17.3 51.8,18.2 Q1.2 52.65,19.2 v53.2,19.2 | C1.2 53.2,18.18 v53.2,19.2 | C14.2 52.3,20.1 v53.2,19.2 | U1.12 33.91,24 v33,24 | U4.4 v23.39,26 v23.4,26 | U1.14 35.12,22.1 v35.5,22.1 | C39.2 63.8,40.02 | C22.1 28.98,19.4 v28.2,19.4 | MIC1.3 59.78,15.4 v58.8,15.4 | MIC1.1 58.6,18.78 v58.4,18.9 | MIC1.2 v58,17.1 | USB-C.A12 25.25,43 USB-C.B1 24.67,43.05 USB-C.P$4 23.67,44.05 USB-C.P$6 | USB-C.A1 30.75,43 USB-C.B12 31.33,43.05 USB-C.P$1 31.68,43.5 USB-C.P$3
  Top 0.25: R2.2 51.05,43.15 v51,43.2 | U2.2 53.2,38.4 52.8,38 52.67,38 C17.2 v52.3,36.6 | 47,26.6 47.2,26.6 v47.2,27.8
  Top 0.3: R13.2 30.66,11.36 v30.7,11.4 | R4.2 21.58,11.98 v21.6,12 | R11.1 15.25,10.55 15.3,10.5 v15.4,10.6 | R1.2 v2.4,6 | R60.2 39.54,9.66 v39.9,9.3 | R61.2 48.82,9.68 v49.3,9.2 | C28.2 44.58,15.72 44.6,15.7 arc60 v44.6,15.6 | v71.8,10.2 71.9,10.1 C3.2 73.2,9.72 73.2,9 74.25,7.95 RST.P2 | C26.2 31.32,28.73 v31.4,28.8 | C21.2 32.9,29.3 v32.2,30 33.1,30.9 C10.1 | C25.2 40.12,31.27 v40.2,31.2 | C19.1 36.7,31.5 v36.6,31.6 | C4.2 v49,23.4 | C33.2 48.58,19.77 v48.4,19.6 | 64.28,22.71 C32.1 63.95,22.8 | 64.28,22.71 64.4,22.6 v65.2,22.6 | v67.2,44.2 67.1,44.3 MICRO_SD.9 67.1,45.9 v67.2,46 | MICRO_SD.10 v56.1,44.1 | RST.P1 RST.P2 | RST.P2 74.45,7.95 v73.95,8.45 | 64.28,22.71 63.83,22.25 C5.2 63.83,20.52 v63.4,20.1
  Top 0.4: 63.8,40.02 v63.8,41 63.75,41.05 MICRO_SD.6
  Top 0.6: C18.2 54.62,42.17 v54.6,42.2 54.5,42.3 R30.2 | TV1.2 v75.4,37.8 | C36.2 v43.8,39.8 | C37.2 46.3,38.8 v46.2,39 | C38.2 50.08,35.73 v50.2,35.6 | C9.2 54.15,28.34 v54.4,28.6 53.55,29.45 C8.2 53.55,29.25 54.4,28.4 | R72.2 v18.4,41.8 | R75.2 19.55,47.95 v19.6,48
  Top 0.67: R12.1 41.05,37.15 v41,37.1
  Top 1: 23.67,44.05 22.15,44.05 v22.1,44.1 | USB-C.P$3 32.55,44.15 v33.7,45.3 | USB-C.P$8 23.7,49 21.9,48.2 v21.8,48.2 | USB-C.P$7 32.33,48.87 v33.8,47.8 | BATT.NEG 62.8,6.6 | 62.8,6.6 61.9,7.5 v61.9,8.45 | 62.8,6.6 64.15,7.95 v64.15,8.5
  pour GND (isolate 0.61): -3.2,52.4 84,52.4 84,-3.8 -3.2,-3.8
GPIO0_3  (via drill 0.3)
  Top 0.2: U1.22 36.6,17.93 36.6,16.6
  Top 0.25: 36.6,16.6 36.7,16.6 v36.8,16.5 | v40.1,13.8 40.3,14 48,14 48.4,13.6 58.4,13.6 58.6,13.4 62.8,13.4 64.4,15 64.4,19.8 69.8,25.2 69.8,27 70.81,28.01 JP2.7
  Top 0.6: JP2.7 72.41,28.01 72.4,28
  Bottom 0.25: v36.8,16.5 37.2,16.5 v40.1,13.8
HP_CBUFF
  Top 0.2: U1.43 43.25,27.4 43.8,27.4 44.2,27.8 44.2,30.8 46.05,32.65 R35.1
  Top 0.3: R35.1 45.25,32.65 45.1,32.8 45.1,43.1 46.5,44.5 48.7,44.5 50.6,46.4
  Top 0.6: HP.5 50.6,46.4
HP_LEFT
  Top 0.2: U1.44 42.94,27.8 43.4,27.8 43.6,28 43.6,31.6 43.8,31.8 R34.1
  Top 0.3: R34.1 43.15,32.65 42.8,33 42.8,41
  Top 0.6: HP.4 42.8,41
HP_RIGHT
  Top 0.2: U1.42 43.55,27 44,27 44.8,27.8 44.8,30.6 45.6,31.4 47.2,31.4 48.4,32.6 R36.1
  Top 0.3: R36.1 47.55,33.65 47.4,33.8 47.4,38.1 HP.1
  Top 0.6: HP.1 48,38.4 47.6,38 47.6,38.2
I2S_12M  (via drill 0.3)
  Top 0.2: U1.21 37.4,19.43 37.4,20.2 v37.3,20.3
  Bottom 0.2: v37.3,20.3 32.4,20.3 31.1,18.9 30.6,18.4 30.6,15.4 29.4,14.2 2.2,14.2 1,15.4 1,23 2,24 3.6,24 3.94,24 JP11.1
  Bottom 0.6: JP11.1 3.71,24.11 3.6,24
IOVDD  (via drill 0.3, 0.4)
  Top 0.2: v38.8,22.4 38.8,24.77 U1.4 35.37,28.2 33.6,28.2 33.2,27.8 33.1,27.7 C26.1 v33.9,27.7 | v41.6,21.6 41.97,21.6 U1.33 43.57,20 46.33,20 C33.1 | U4.7 U4.8 27.47,17.52 C22.2 | U4.3 24.66,26.64 v24.2,27.1 | R100.2 27.15,28.15 v27.2,28.1
  Top 0.25: R37.1 54.95,48.35 55,48.4 55,49 v54.9,49.1
  Top 0.3: C22.2 v29.1,16.3 | R97.2 24.85,13.3 v25.7,13.3 | R96.2 v29.1,12.8 | LED2.A v4.4,6 | R83.2 37.15,12.25 v36.8,12.6 | R82.2 v44.7,10.5 | R101.2 22.05,25.55 v22.4,25.8 | C33.1 46.1,20.3 v46,20.2 | R24.2 67.45,13.15 v67.4,13.2 | R3.2 67.25,19.05 v67.2,19
  Top 0.6: R8.2 63.5,27.1 v63.4,27 | v33.9,27.7 33.8,27.8 33.2,27.8
  Bottom 0.2: v38.8,22.4 39.6,21.6 v41.6,21.6
  pour VCC (isolate 0.61): -1.2,50.8 82.8,50.8 82.8,-2.2 -1.2,-2.2 -1.2,50.6
LED1  (via drill 0.3, 0.4)
  Top 0.2: 36.19,26 U1.6 35.3,26.85 v35.3,27.2 | v50.2,34 52.2,34 52.8,34.6 57.4,34.6 59,36.2 69.8,36.2 71.6,34.4 74.46,34.4 JP2.4
  Top 0.25: v35,34.3 40,34.3 v40.9,35.2 | LD.A 53.2,45.6 v53.3,45.5
  Top 0.6: JP2.4 75.77,33.23 75.2,33.8
  Bottom 0.2: 48.2,35.8 48.4,35.8 v50.2,34
  Bottom 0.25: v35.3,27.2 35.3,34 v35,34.3 | v40.9,35.2 47.6,35.2 48.2,35.8 50.4,38 50.4,40.4 52.6,42.6 52.6,44.8 v53.3,45.5
MISO0
  Top 0.2: R100.1 26,23.88 U4.2 25.93,22.27 | U1.8 34.34,26.4 29.6,26.4 28.4,25.2 28.4,22.2 28,21.8 26.4,21.8 25.93,22.27 | 25.93,22.27 25.47,21.8 22.6,21.8 20.19,24.21 JP5.2
  Top 0.6: JP5.2 18.79,24.21 18.8,24.2
MISO1  (via drill 0.3, 0.4)
  Top 0.2: U1.16 34,19.57 34,18.4
  Top 0.25: v42.8,11.3 43.1,11.3 43.4,11.6 69,11.6 v70.8,13.4 | v70.7,17.5 70.7,19.1 72,20.4 72.4,20.4 | 73.2,20.4 JP2.13
  Top 0.3: 34,18.4 v34.1,18.5
  Top 0.6: 72.4,20.4 73.2,20.4
  Bottom 0.25: 34.4,12.8 35.8,11.4 42.7,11.4 v42.8,11.3 | v70.8,13.4 70.8,17.4 v70.7,17.5
  Bottom 0.3: v34.1,18.5 34.4,18.2 34.4,12.8
MOSI0  (via drill 0.4)
  Top 0.2: U4.5 23.39,19.8 24,20.4 30.2,20.4 30.4,20.2 30.4,16.6 31.2,15.8 38,15.8 38.6,16.4 39.2,16.99 U1.25 | U4.5 23.39,19.8 22.8,20.4 20.4,20.4 19.2,21.6 18.8,21.6 18.44,21.6 JP5.4 | U4.5 23.39,13.01 24.4,12 26,12 27.8,10.2 29.05,10.2 R96.1 29.5,9.75
  Top 0.3: B2.P1 B2.P2 29.73,8.08 29.73,8.18 | 29.73,8.18 29.15,8.75 29.15,10.1 R96.1 | 29.73,8.18 29.73,8.22 v29.45,8.5
  Top 0.6: JP5.4 18.73,21.67 18.8,21.6
MOSI1  (via drill 0.3, 0.4)
  Top 0.2: U1.15 33.4,19.68 v33.4,17.6
  Top 0.25: v33.4,14.2 33.8,14.2 34.2,14.6 48.4,14.6 48.8,14.2 53.6,14.2 54.6,15.4 54.6,19.8 53.8,20.6 v53.8,22 | v56.4,26.6 RP1.6
  Bottom 0.2: v53.8,22 56.2,19.6 59,19.6 62.4,23 63.4,23 65.4,25 68.4,25 69.2,24.2 74.6,24.2 75.2,23.6 | 75.77,23.03 JP2.12
  Bottom 0.25: v53.8,22 53.8,24 v56.4,26.6
  Bottom 0.3: v33.4,17.6 v33.4,14.2
  Bottom 0.6: 75.77,23.03 75.2,23.6
N$2  (via drill 0.3)
  Top 0.25: LD.C 52.85,48.55 v52.4,49 | R2.1 50.85,44.85 v50.7,44.7
  Bottom 0.25: v52.4,49 50.8,49 49.2,47.4 49.2,46.2 v50.7,44.7
N$3
  Top 0.3: LED2.C 2.6,2.75 R1.1
N$5
  Top 0.25: JP9.3 34.2,43.74 34.2,43.2 33.4,42.4 33.4,40.1 34.7,38.8 34.7,38.3 RP3.5
  Top 0.6: JP9.3 36.27,45.87 35.6,45.2
N$6  (via drill 0.4)
  Top 0.3: R60.1 42.27,9.43 B1.S2 | B1.S1 B1.S2 | B1.S2 42.27,8.62 v42.25,8.65
N$7
  Top 0.25: 35.4,43.2 34.2,42 34.2,40.2 35.6,38.8 RP3.3
  Top 0.6: JP9.5 35.4,43.2
N$8
  Top 0.25: MIC1.5 62.07,17.2 61.4,17.2 60.9,17.7 60.9,19.6 60.2,20.3 60.2,22.8 59.13,23.87 JP1.2
N$9  (via drill 0.4)
  Top 0.3: 14.2,8.4 14.4,8.2 14.32,8.12 PWR.S2 PWR.S1 | 14.2,8.4 12.8,9.8 12.8,10.4 12.65,10.4 R10.2 10.62,10.65 C2.2 | 14.2,8.4 14.2,8.45 v14.15,8.5
N$10
  Top 0.2: U1.41 43.86,26.6 45.2,26.6 45.4,26.8 C27.1
N$11
  Top 0.2: 58.6,14.4 57.2,15.8 57.2,19 58.6,20.4 58.6,21.16
  Top 0.25: JP1.4 58.6,21.16 | 58.6,14.4 59,14 60.6,14 62.05,15.45 MIC1.4
N$12
  Top 0.2: RP1.1 65.5,29.3 67.4,31.2 67.4,31.6 JP7.2
  Top 0.6: JP7.2 67.41,31.61 67.4,31.6
N$13
  Top 0.2: RP1.5 56.4,30.2 56.8,30.6 61.4,30.6 62.33,31.53 JP7.6
  Top 0.6: JP7.6 62.33,31.73 62.2,31.6
N$14  (via drill 0.5)
  Top 0.3: R14.2 69.45,38.25 v69.4,38.2
  Bottom 0.3: JP7.7 JP7.5 JP7.3 JP7.1 68.47,34.87
  Bottom 0.6: JP7.7 68.47,34.87 69.4,35.8 v69.4,38.2
N$15
  Top 0.2: RP1.3 57.2,30 57.4,30.2 58.8,30.2 59.2,29.8 63.4,29.8 64.87,31.27 JP7.4
  Top 0.6: JP7.4 64.87,31.67 64.8,31.6
N$16
  Top 0.2: RP1.7 55.6,30.2 56.8,31.4 58.86,31.4 JP7.8
  Top 0.6: JP7.8 59.73,32.33 59.2,31.8
N$17
  Top 0.3: R34.2 C36.1
N$18
  Top 0.6: R7.1 74.25,42.05 VIDEO.2
N$19
  Top 0.2: C38.1 48.33,35.42 R36.2
N$20
  Top 0.3: R35.2 C37.1
N$21
  Top 0.25: MICRO_SD.12 54.95,46.6 R37.2
N$25
  Top 0.25: JP9.1 36.39,48.41 37.6,47.2 37.6,42.5 37.2,42.1 35.5,42.1 34.9,41.5 34.9,40.2 35.8,39.3 36,39.3 36.4,38.9 RP3.1
N$41  (via drill 0.4)
  Top 0.3: R61.1 51.22,9.77 51.17,9.72 B0.S2 | B0.S1 B0.S2 | B0.S2 51.17,8.68 v51.2,8.7
N$48
  cutout Top: 1.3,9.2 1.3,7.2 6.3,7.2 6.3,9.2
  cutout GND: 1.3,9.2 1.3,7.2 6.3,7.2 6.3,9.2
  cutout VCC: 1.3,9.2 1.3,7.2 6.3,7.2 6.3,9.2
N$52
  Top 0.3: R14.1 R7.2 72.55,37.9 TV1.1
N$89  (via drill 0.4)
  Top 0.3: 33.5,9.1 33.48,9.12 | 33.48,9.12 R13.1 | B2.S1 B2.S2 | B2.S2 33.48,9.12 | B2.S2 33.48,8.68 v33.5,8.7
N$100  (via drill 0.4)
  Top 0.3: R4.1 24.3,9.74 v24.3,8.6 24.3,8.35 24.3,8.2 24.32,8.18 B3.S2 B3.S1
PWRB  (via drill 0.4)
  Top 0.2: U1.5 37.4,25.46 37.4,24.2 36,22.8 30.4,22.8 28.4,20.8 22,20.8 21.4,21.4 v20.6,21.4 | v20.6,18 20.6,15.2 17.65,12.25 R11.2 14.3,12.35 R10.1
  Bottom 0.2: v20.6,21.4 v20.6,18
Q1N
  Top 0.2: U1.31 42.75,19.4 46.6,19.4 47.65,18.35 R6.2 | 48.25,18.35 R6.2 | R6.2 Q1.3 50.12,18.48 C14.1
Q1P
  Top 0.2: U1.30 42.45,19 46,19 48.35,16.65 R6.1 48.6,16.45 48.6,15.4 49.2,14.8 51.2,14.8 51.8,15.4 Q1.1 51.88,16.12 C1.1
RTCVDD  (via drill 0.3, 0.4)
  Top 0.2: U1.37 44.29,24.2 45.4,24.2 46.12,23.48 C4.1 | D6.CATHODE 53.8,6.74
  Top 0.3: C4.1 46.12,23.93 46.6,24.4 50,24.4 v50.4,24 | v55.4,17.8 55.4,17.2 56.2,16.4 56.2,14.8 v56.6,14.4 | 53.8,6.74 54.15,6.74 | 54.15,6.74 56.06,6.74 BATT.P2 | v54.95,8.35 54.95,7.5 54.45,7 54.41,7 54.15,6.74
  Bottom 0.3: v50.4,24 52.2,22.2 52.2,21.4 54.2,19.4 54.2,19 v55.4,17.8 | v56.6,14.4 56.6,10 v54.95,8.35
  Bottom 1: BATT.P2 BATT.P1
RX0  (via drill 0.4)
  Top 0.2: U1.19 35.2,18.65 v35.2,16.6
  Top 0.25: v35.3,13.7 35.4,13.8 38.8,13.8 39.6,13 58.2,13 58.4,12.8 64,12.8 | 74.6,16.6 75.2,17.2 75.8,17.8 76,17.8 75.95,17.85 JP2.16
  Top 0.3: 64,12.8 64.4,12.8 67.6,16 67.6,16.75 R3.1 68.95,16.6 74.6,16.6
  Top 0.6: JP2.16 75.2,17.28 75.2,17.2
  Bottom 0.25: v35.2,16.6 35.2,13.8 v35.3,13.7
RX1  (via drill 0.3, 0.4)
  Top 0.2: JP2.5 71.15,30.55 68,27.4 66.35,27.4 R8.1 66.05,26.65 65.2,25.8 55.8,25.8 51.6,21.6 45.2,21.6 44.6,21 43.98,21 U1.35 42,22.98 v42,23
  Top 0.25: RP3.4 35.6,36.2 36,35.6 36.4,35.3 v37.3,35.3
  Top 0.6: JP2.5 72.45,30.55 72.4,30.6
  Bottom 0.2: 42,23.18 v42,23
  Bottom 0.25: 42,23.18 42,24.6 38.6,28 38.6,34 v37.3,35.3
SCK0  (via drill 0.4)
  Top 0.2: U1.27 41.8,17.52 41.8,16.6 40.35,15.15 v26.2,15.15 R97.1 24.66,15.19 U4.6 | 20.3,13.5 v22,15.2 21.6,15.6 21.6,18.6 21.07,19.13 JP5.6
  Top 0.3: B3.P1 B3.P2 20.57,8.28 20.55,8.3 v20.25,8.6 20.15,8.7 20.15,13.35 20.3,13.5
  Top 0.6: JP5.6 18.73,19.13 18.8,19.2
  Bottom 0.2: v22,15.2 26.15,15.2 v26.2,15.15
SCK1  (via drill 0.4)
  Top 0.2: U1.17 37.6,22.46 v37.6,22.8 | v66,17 66,19.6 68.2,21.8 v70.8,21.8
  Bottom 0.2: v37.6,22.8 37.6,22.2 38.4,21.4 38.4,17.8 40,16.2 41.4,16.2 43.6,18.4 50.8,18.4 53,16.2 65.2,16.2 v66,17 | v70.8,21.8 71.9,21.8 72.1,21.6 75.1,21.6 75.7,21 75.7,20.46 JP2.14
  Bottom 0.6: 75.7,20.46 75.7,20.9 75.4,21.2
SD_CLK  (via drill 0.4)
  Top 0.2: U1.24 38.69,18.6 v39.1,18.6 | MICRO_SD.5 62.7,42.55 v62.7,41.2
  Bottom 0.2: v39.1,18.6 42.2,18.6 54,30.4 54,33.2 58.4,37.6 61.8,37.6 62.8,38.6 62.8,40.8 62.7,40.9 v62.7,41.2
SD_CMD  (via drill 0.4)
  Top 0.2: U1.23 38.6,19.22 v39.2,19.8 | v60.4,38.8 60.45,38.85 R17.1 MICRO_SD.3
  Bottom 0.2: v39.2,19.8 39.8,19.2 42,19.2 53.4,30.6 53.4,33.4 58.2,38.2 60,38.2 60.4,38.6 v60.4,38.8
SD_DAT0  (via drill 0.4)
  Top 0.2: U1.26 41,17.62 v41,17 | MICRO_SD.7 64.85,40.95 65.2,40.6 65.2,39.85 R15.1 65.25,38.65 v65.2,38.6
  Bottom 0.2: v65.2,38.6 65.2,38.4 63.8,37 58.6,37 54.6,33 54.6,30.2 41.4,17 v41,17
SD_PWR_RST
  Top 0.25: U2.3 53.95,37.4 55,37.4 55.2,37.6 55.2,40 55,40.2 53.8,40.2 53.4,40.6 53.4,43.8 54.35,44.75 R30.1 54.95,45.2 55,45.2 55.3,45.5 MICRO_SD.11
SPDIFI  (via drill 0.3, 0.4)
  Top 0.2: U1.9 35.8,24.23 v35.8,23.6 | RP1.4 57.2,26.9 v57.6,26.5
  Top 0.3: v20,27.7 14.1,27.7 12.4,26 3,26 2,25 2,22 2.4,21.6 3.46,21.6 JP11.3
  Top 0.6: JP11.3 3.63,21.57 3.6,21.6
  VCC 0.2: v35.8,23.6 36.6,23.6 37.2,24.2 39,24.2 39.2,24 44.8,24 46.6,22.2 50.4,22.2 52.1,23.9 56.2,23.9 JP1.1
  Bottom 0.2: JP2.9 64.87,25.47 63,23.6 61.8,23.6 60.8,24.6 60.8,26.4 59.8,27.4 58.6,27.4 57.7,26.5 v57.6,26.5 57.6,26.2 56.2,24.8 56.2,23.9 JP1.1
  Bottom 0.3: v35.8,23.6 35.8,24.4 33.8,26.4 31.6,26.4 28,30 22,30 21.4,29.4 21,29.4 20.2,28.6 20.2,27.9 v20,27.7
  Bottom 0.6: JP2.9 72.47,25.47 72.4,25.4
SPDIFO  (via drill 0.3, 0.4)
  Top 0.2: U1.10 33.73,25.6 v33,25.6 | RP1.2 58,27.5 v58.9,26.6 61.6,26.6 63.4,28.4 67.8,28.4 v68.7,29.3
  Top 0.3: v21.9,28.6 14,28.6 12.6,27.2 3,27.2 1,25.2 1,20.2 2.2,19 3.4,19 3.6,19 JP11.5
  Top 0.6: JP11.5 3.43,19.03 3.4,19
  VCC 0.2: JP1.3 42.87,21.33 42,22.2 40.2,22.2 38.8,23.6 37.2,23.6 36.4,22.8 35.4,22.8 34.8,23.4 34.8,23.8 v33,25.6
  Bottom 0.2: JP1.3 57.5,22.6 57.5,24.6 58.7,25.8 58.7,26.4 v58.9,26.6 | v68.7,29.3 74.48,29.3 JP2.8
  Bottom 0.3: v33,25.6 31.4,25.6 27.6,29.4 22.7,29.4 v21.9,28.6
  Bottom 0.6: JP2.8 75.59,28.01 75.2,28.4
SPK0  (via drill 0.3, 0.4)
  Top 0.2: v43.2,22.8 43.2,22.49 U1.36 44.54,21.74 44.8,22 50.7,22 v53.4,24.7 | v60.1,28.4 60.4,28.4 60.8,28.8 66.6,28.8 70.89,33.09 JP2.3
  Top 0.25: v38.5,35.7 37.6,36.6 | 37.6,36.6 RP3.2 | 37.6,36.6 39.35,38.35 R12.2 39.35,38.45 38.8,39 38,39 37.2,39.8
  Top 0.6: JP2.3 72.29,33.09 72.2,33
  Top 0.67: JP9.7 36.33,40.67 37.2,39.8
  Bottom 0.2: v53.4,24.7 53.5,24.7 55,26.2 55,27 56.4,28.4 v60.1,28.4
  Bottom 0.25: v43.2,22.8 43.2,24.2 39.2,28.2 39.2,35 v38.5,35.7
TX0  (via drill 0.3)
  Top 0.2: U1.20 35.9,18.64 v35.9,17.4
  Top 0.25: 35.8,17.2 v35.9,17.4 | v39.5,12.3 39.6,12.2 64.6,12.2 67.25,14.85 R24.1 68.76,15.31 JP2.17
  Top 0.6: JP2.17 73.14,15.4 72.4,15.4
  Bottom 0.2: 36,17.2 36,17.3 v35.9,17.4
  Bottom 0.25: v35.9,17.4 36,17.4 | 36,17.2 36,15.2 37.2,14 37.8,14 v39.5,12.3
TX1  (via drill 0.3, 0.4)
  Top 0.2: v40.8,23.2 41.7,22.3 41.98,22.3 U1.34 43.67,20.6 45,20.6 45.6,21.2 51.8,21.2 56,25.4 68.6,25.4 69.2,26 69.2,27.4 71.1,29.3 74.5,29.3 75.2,30
  Top 0.25: RP3.6 34.8,35.8 35.2,35.2 v35.5,35
  Top 0.6: JP2.6 75.75,30.55 75.2,30
  Bottom 0.25: v40.8,23.2 40.8,25 37.8,28 37.8,33.2 v35.5,35
USB2+
  Bottom 0.2: 11.65,34.95 10.8,35.8 10.8,37.8 10.2,38.4 8.4,38.4 7.6,37.6 X2.3
  Bottom 0.3: 11.65,34.95 18.4,34.95 SW1.12 | X2.3 7.6,37.55 7.85,37.8
USB2-
  Bottom 0.2: 18.88,33.12 18,34 10.8,34 9.6,35.2 9.6,36.1
  Bottom 0.3: SW1.22 19,33 18.88,33.12 | X2.2 9.6,36.1
VH1  (via drill 0.4)
  Top 0.2: U1.2 36.7,28.28 C19.2 36.02,30.1 C10.2
  Top 0.3: C10.2 34.88,31.73 34.7,31.9 31.9,31.9 30.4,30.4 29.8,30.4 29,29.6 14,29.6 12.6,28.2 7.4,28.2 6.07,29.53 JP8.1 | 10.5,8.1 10.57,8.03 PWR.P2 PWR.P1 | 10.5,8.1 9.2,9.4 9.2,11.8 9.8,12.4 10.57,12.4 C2.1 10.6,14 9.8,14.8 v9.8,25.1 | 10.5,8.1 10.5,8.2 v10.3,8.4
  Bottom 0.3: v9.8,25.1 9.8,28.07 JP8.1
VHIGH  (via drill 0.5)
  Top 0.2: USB-C.B4 26.75,43 USB-C.A9 26.75,40.95 26.4,40.6 | USB-C.B9 29.25,43 USB-C.A4 29.25,40.95 29.6,40.6
  Top 0.25: U2.1 52.33,39.35 C17.1
  Top 0.3: 26.4,40.6 25.4,40.6 v22.6,37.8 21.8,37.8 21.76,37.76 | 29.6,40.6 29.6,38.8 | 29.6,38.8 27.4,36.6 v25.6,36.6 | 29.6,38.8 v32,38.8 | v49.4,40.4 51.27,40.4 C17.1 51.38,39.38 51.2,39.2 51.2,36 52,35.2 57.2,35.2 58.8,36.8 70.4,36.8 71.6,35.6 72.4,35.6 73.2,35.6 JP2.1
  Top 0.6: X2.1 12.1,35.3 11.4,34.6 | 11.4,34.6 11,34.2 11,31.87 JP3.2 | 21.76,37.76 18.56,37.76 15.4,34.6 11.4,34.6 | JP2.1 72.43,35.63 72.4,35.6
  Bottom 0.3: v25.6,36.6 23.8,36.6 v22.6,37.8 | v32,38.8 44,38.8 45.6,40.4 v49.4,40.4
  Bottom 0.6: 11,31.87 JP3.2 10.8,31.8 8.2,34.4 4.2,34.4 3.6,33.8 3.6,31.87 JP8.2
XCS0  (via drill 0.3, 0.4)
  Top 0.2: 29.2,26.8 27.2,24.8 U4.1 | 29.2,26.8 34.65,26.8 U1.7 36.6,24.85 v36.6,24.6 | 29.2,26.8 28.2,27.8 28.2,28.6 27.8,29 23.8,29 22.2,27.4 21.25,27.4 R101.1 21.15,27.35 20.4,26.6 15,26.6 13.6,25.2 13.6,17.19 14.2,16.59 JP5.7 | JP2.10 74.5,24.2 69.7,24.2 65.1,19.6 v65.1,15.3
  Top 0.6: JP5.7 14.61,16.59 14.6,16.6 | JP2.10 75.67,25.47 75.2,25
  Bottom 0.2: v36.6,24.6 36.6,24.2 36.8,24 36.8,22.2 38,21 38,17.6 39.8,15.8 41.6,15.8 43.8,18 50.4,18 53,15.4 57.2,15.4 58.6,14 63.8,14 v65.1,15.3
XCS1  (via drill 0.3, 0.4)
  Top 0.2: U1.18 37.45,21.6 38.6,21.6 39.1,21.1 v39.1,21 | v44.4,22.8 44.8,22.4 50,22.4 52,24.4 | 52,24.4 53,25.4 54.6,25.4 55.6,26.4 RP1.8 | v51.6,24.6 51.8,24.6 52,24.4
  Bottom 0.2: v39.1,21 40.3,19.8 41.4,19.8 v44.4,22.8 | JP2.15 73.15,17.85 | 72.6,18.4 66.6,24.4 65.6,24.4 63.6,22.4 62.4,22.4 60.8,20.8 60.8,19.2 59.8,18.2 56.4,18.2 52.8,21.8 52.8,23.4 v51.6,24.6
  Bottom 0.6: 73.15,17.85 72.6,18.4
XHLD0  (via drill 0.3, 0.4)
  Top 0.2: U1.28 42.6,17.43 42.6,15.8 42.3,15.5 v42.2,15.5 | JP11.4 7,21.6 | 7.8,21.6 8,21.6 8.5,21.1 v8.5,5.2
  Top 0.3: R82.1 47.35,9.55 v47.4,9.5 47.4,9.2 47.38,8.68 B0.P2 | B0.P1 47.42,2.33 47.7,2.6 v45.6,4.7 45.6,5.2 47.4,7 47.4,7.97 B0.P2 | B0.P2 v47.4,8.7
  Top 0.6: 7,21.6 7.8,21.6
  Bottom 0.2: v42.2,15.5 47.4,10.3 v47.4,9.5 | v8.5,5.2 9,4.7 v45.6,4.7
  Bottom 0.3: JP5.5 12.07,19.13 9.6,21.6 7.8,21.6 | 7,21.6 6.8,21.6 JP11.4
  Bottom 0.6: 7,21.6 7.8,21.6 | JP5.5 14.67,19.13 14.6,19.2
XRST  (via drill 0.4)
  Top 0.2: U1.13 32.4,20.09 v32.4,16.8
  Top 0.3: v32.4,13 35,10.4 35,8.6 36.2,7.4 36.2,1.2 36.8,0.6 77,0.6 77.6,1.2 77.6,1.32 | 77.6,1.32 77.9,1.5 | C3.1 R28.1 76.4,9.95 76.5,9.6 78.15,7.95 RST.S2 | 77.6,1.32 RST.S1 RST.S2 | RST.S2 78.22,7.97 v77.7,8.5
  Bottom 0.3: v32.4,16.8 v32.4,13
XTALI_RTC
  Top 0.2: U1.39 44.08,25.4 47.6,25.4 51.15,28.95 Q7.2 51.8,29.16 C8.1
XTALO_RTC
  Top 0.2: U1.38 44.38,25 47.8,25 49.25,26.45 Q7.1 51.73,26.59 C9.1
XWP0  (via drill 0.3, 0.4)
  Top 0.2: U1.11 33.82,24.8 31.8,24.8 v31.45,24.45 28.4,21.4 22.2,21.4 20.7,22.9 16.6,22.9 16.2,22.5 15.6,21.84 JP5.3 | 38.5,8.25 v38.15,8.6 37.4,9.35 37.4,10.25 R83.1 35.85,10.55 32.2,14.2 v31.4,14.2 | v31.6,17.8 31.6,21.7 v31.5,22
  Top 0.3: B1.P1 B1.P2 | B1.P2 38.52,8.28 38.5,8.25 | B1.P2 38.52,8.22 v38.15,8.6
  Top 0.6: 15.6,21.84 15.6,22 16,22.4
  Bottom 0.2: v31.4,14.2 31.4,14.6 31.6,14.8 v31.6,17.8 | v31.5,22 31.5,24.4 v31.45,24.45
  Bottom 0.3: JP5.3 15.2,21.67 12.73,21.67 10.1,24.1 6.76,24.1 JP11.2
  Bottom 0.6: JP11.2 7.89,24.11 8,24 | 15.2,21.67 14.67,21.67 14.6,21.6

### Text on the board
Top: 1
GND: 2
VCC: 3
Bottom: 4
tPlace: S2/11 | G | S0 | G | S1 | G | A<->C | S2 | G | 5V | IOV | 5v | Vhigh | 5v | GND | SPK0 | LD1 | SPI | RX1 | CS1 | MOSI1 | SPO | TX1 | GPIO0_3 | SPO | I2S | FLASH | mic | SPDIFI | CS0 | 12M | BCK | IOV | MISO | clock | CVDD | DI | WP0 | data | MO / SI1 | FRM | MOSI | MISO1 | DO | HLD0 | sck1 | IOV | SCK0 | CS1 | GND | CS0 | RX0 | GND | GND | TX0 | AVD | VS1010 LQFP simple board | GND | GND | V1.20 / 3/2021 PL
